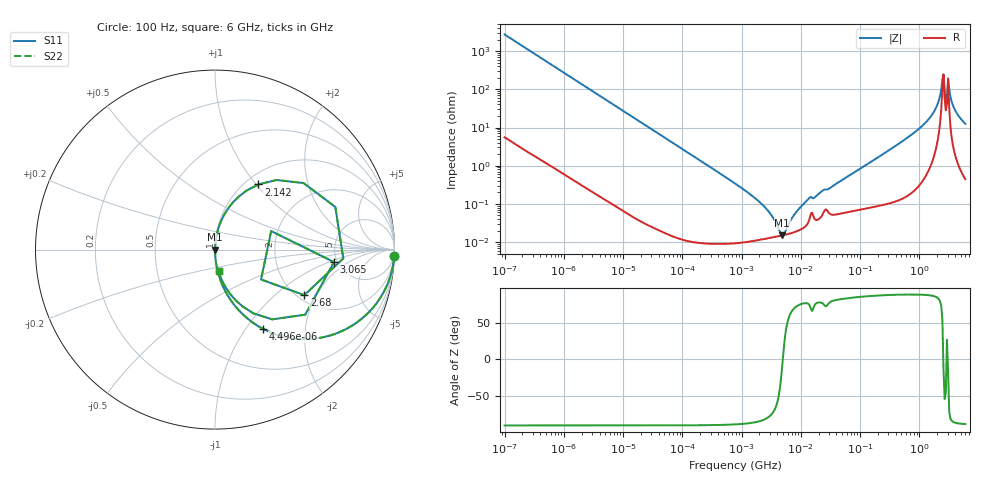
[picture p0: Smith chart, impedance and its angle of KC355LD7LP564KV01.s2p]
!Murata Part Number: KC355LD7LP564KV01
!These Parameters are Measured in Series Mode Connection
!Data Generated on Jun 19, 2026
!  o--ll--o
!Port1  Port2
!  o------o
!Operation Temp=25[degC], DC Bias Voltage=0[V]
!Freq. Start=100[Hz] Stop=6[GHz] 401[Steps]
# Hz S RI R 50
!Freq.(Hz) S11(Real) S11(Imag) S21(Real) S21(Imag) S12(Real) S12(Imag) S22(Real) S22(Imag)
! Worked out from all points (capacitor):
!   401 points, 100 Hz to 6 GHz, reference 50 ohm
!   read as one part in series: C = 586 nF near 109 Hz
!   lowest |Z| = 15.2 mohm at 4.857 MHz (marker M1)
!   series resonance near 4.96 MHz, so ESL is about 1.8 nH
!   S11 on the Smith chart (normalised r, x): 100 Hz: 1, -54; 4.496 kHz: 1.00, -1.21; 2.142 GHz: 1.15, +1.03; 2.68 GHz: 2.17, -1.60; 3.065 GHz: 4.69, -1.17; 6 GHz: 1.01, -0.25
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100  0.9986 -0.0368  0.00143 0.0368  0.00143 0.0368  0.9986 -0.0368
686  0.9399 -0.2366  0.0601 0.2366  0.0601 0.2366  0.9399 -0.2366
2008  0.6479 -0.4765  0.3521 0.4765  0.3521 0.4765  0.6479 -0.4765
4496  0.2698 -0.4427  0.7302 0.4427  0.7302 0.4427  0.2698 -0.4427
10527  0.0637 -0.2429  0.9363 0.2429  0.9363 0.2429  0.0637 -0.2429
40335  0.00479 -0.0675  0.9952 0.0675  0.9952 0.0675  0.00479 -0.0675
774597  0.000105 -0.00344  0.9999 0.00344  0.9999 0.00344  0.000105 -0.00344
2481164  0.000123 -0.000811  0.9999 0.000811  0.9999 0.000811  0.000123 -0.000811
4856642  0.00015 -2.22e-05  0.9998 2.22e-05  0.9998 2.22e-05  0.00015 -2.22e-05
8692127  0.000196 0.000632  0.9998 -0.000632  0.9998 -0.000632  0.000196 0.000632
1.555665e7  0.000588 0.00131  0.9994 -0.00131  0.9994 -0.00131  0.000588 0.00131
3.124326e8  0.0017 0.0257  0.9983 -0.0257  0.9983 -0.0257  0.0017 0.0257
1.197065e9  0.0188 0.1186  0.9812 -0.1186  0.9812 -0.1186  0.0188 0.1186
1.791126e9  0.0816 0.2408  0.9184 -0.2408  0.9184 -0.2408  0.0816 0.2408
2.142435e9  0.2417 0.363  0.7583 -0.363  0.7583 -0.363  0.2417 0.363
2.450438e9  0.6703 0.2376  0.3297 -0.2376  0.3297 -0.2376  0.6703 0.2376
2.679998e9  0.4978 -0.2537  0.5022 0.2537  0.5022 0.2537  0.4978 -0.2537
3.065283e9  0.6631 -0.0695  0.3369 0.0695  0.3369 0.0695  0.6631 -0.0695
3.352442e9  0.319 -0.3887  0.681 0.3887  0.681 0.3887  0.319 -0.3887
3.505958e9  0.2151 -0.3555  0.7849 0.3555  0.7849 0.3555  0.2151 -0.3555
4.193612e9  0.0717 -0.2295  0.9283 0.2295  0.9283 0.2295  0.0717 -0.2295
6e9  0.0195 -0.1217  0.9805 0.1217  0.9805 0.1217  0.0195 -0.1217
